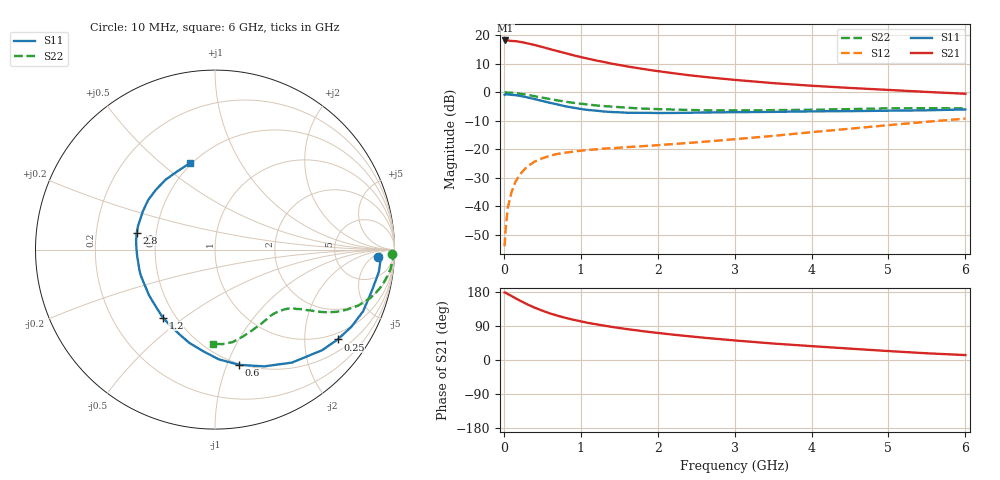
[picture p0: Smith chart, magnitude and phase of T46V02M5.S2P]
! Infineon Technologies  Discrete & RF Semiconductors
! BFR182T
! Si NPN RF Bipolar Junction Transistor in SC75
! VCE = 6 V  IC = 2.5 mA
! Common Emitter S-Parameters:  October  1999
# GHz  S  MA  R  50
!  f  S11  S21  S12  S22
! GHz  MAG  ANG  MAG  ANG  MAG  ANG  MAG  ANG
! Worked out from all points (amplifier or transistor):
!   36 points, 10 MHz to 6 GHz, reference 50 ohm
!   highest |S21| = 18.2 dB at 20 MHz (marker M1)
!   |S21| within 3 dB of that: start of sweep to 594.4 MHz
!   unconditionally stable (mu >= 1): 1.89 GHz to 4.308 GHz
!   at 250 MHz: K = 0.17, MSG = 22.5 dB, |S12| = -27.6 dB
!   at 1.4 GHz: K = 0.82, MSG = 14.9 dB, |S12| = -19.6 dB
!   at 6 GHz: K = 0.83, MSG = 4.4 dB, |S12| = -9.2 dB
!   lowest NFmin = 1.10 dB at 450 MHz
!   S11 on the Smith chart (normalised r, x): 10 MHz: 17, -8; 250 MHz: 0.80, -2.86; 600 MHz: 0.49, -1.11; 1.2 GHz: 0.43, -0.42; 2.8 GHz: 0.39, +0.09; 6 GHz: 0.49, +0.63
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0.01  0.9092 -2.6  8.1 178.0  0.002 84.1  0.9879 -1.4
0.02  0.9267 -1.8  8.147 177.9  0.0035 96.2  0.9999 -1.4
0.05  0.9214 -7.7  8.116 174.2  0.0093 86.0  0.9915 -3.2
0.1  0.9038 -14.6  8.001 169.0  0.0178 83.7  0.9843 -6.3
0.15  0.8939 -22.6  7.91 163.1  0.0267 76.9  0.9685 -9.3
0.25  0.8474 -36.2  7.521 152.5  0.0419 70.0  0.9299 -14.8
0.3  0.8188 -43.2  7.278 147.4  0.0493 68.0  0.9078 -17.2
0.4  0.7618 -55.7  6.782 138.1  0.061 62.0  0.8566 -21.4
0.5  0.7063 -67.1  6.251 130.2  0.0697 57.0  0.8085 -24.4
0.6  0.6561 -78.1  5.74 122.9  0.0774 53.1  0.7632 -27.0
0.8  0.5698 -96.7  4.879 111.3  0.0875 48.6  0.687 -30.4
0.9  0.539 -105.4  4.493 106.4  0.091 46.6  0.6562 -31.6
1.1  0.4904 -120.7  3.889 97.7  0.0981 44.5  0.61 -33.5
1.2  0.4776 -127.5  3.624 94.3  0.0998 44.3  0.5898 -34.3
1.4  0.4518 -140.1  3.198 87.5  0.1045 44.1  0.5632 -36.0
1.6  0.4394 -151.5  2.857 81.5  0.1095 44.8  0.5388 -37.4
2.2  0.4352 -175.4  2.172 66.9  0.124 48.6  0.4995 -43.0
2.8  0.4458 167.8  1.759 55.2  0.1429 52.8  0.4816 -49.9
3.5  0.4548 152.5  1.453 43.5  0.1724 56.8  0.4874 -58.5
4.5  0.4683 134.8  1.196 30.0  0.2305 58.6  0.5086 -72.2
5.5  0.4845 115.3  1.018 17.7  0.305 56.2  0.5283 -85.4
6  0.5018 105.9  0.945 13.0  0.3462 53.4  0.5253 -91.2
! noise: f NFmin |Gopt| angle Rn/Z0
0.45  1.1  0.39  29  0.35
0.9  1.2  0.37  59  0.28
1.8  1.8  0.28  128  0.2
